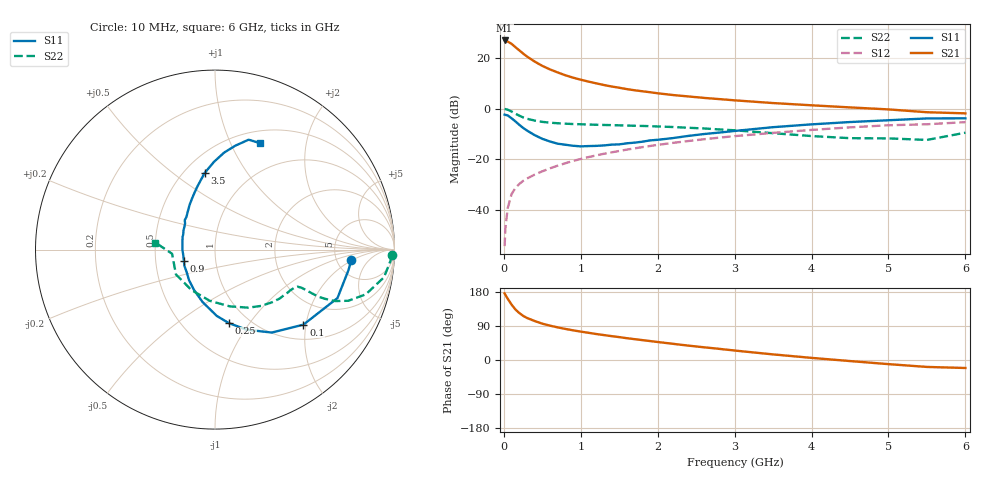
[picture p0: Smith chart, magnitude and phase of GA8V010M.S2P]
! Infineon Technologies  Discrete & RF Semiconductors
! BF775
! Si NPN RF Bipolar Junction Transistor in SOT23
! VCE = 8 V  IC = 10 mA
! Common Emitter S-Parameters:  May  1996
# GHz  S  MA  R  50
!  f  S11  S21  S12  S22
! GHz  MAG  ANG  MAG  ANG  MAG  ANG  MAG  ANG
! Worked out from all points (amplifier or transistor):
!   36 points, 10 MHz to 6 GHz, reference 50 ohm
!   highest |S21| = 27.0 dB at 10 MHz (marker M1)
!   |S21| within 3 dB of that: start of sweep to 164.1 MHz
!   unconditionally stable (mu >= 1): 623.1 MHz to 2.845 GHz
!   at 250 MHz: K = 0.66, MSG = 25.2 dB, |S12| = -28.6 dB
!   at 1.4 GHz: K = 1.09, MAG = 11.2 dB, |S12| = -17.3 dB
!   at 6 GHz: K = 0.89, MSG = 1.7 dB, |S12| = -5.3 dB
!   S11 on the Smith chart (normalised r, x): 10 MHz: 6.85, -1.86; 100 MHz: 1.35, -1.94; 250 MHz: 0.81, -0.80; 900 MHz: 0.70, -0.09; 3.5 GHz: 0.63, +0.65; 6 GHz: 0.64, +1.29
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0.01  0.7608 -4.3  22.35 175.8  0.0019 88.3  0.9876 -1.8
0.02  0.7528 -8.6  21.92 171.9  0.0042 84.3  0.9791 -3.8
0.05  0.7338 -21.6  21.27 161.8  0.0107 80.4  0.9541 -9.3
0.1  0.6462 -40.3  19.17 146.3  0.0203 71.3  0.8768 -16.5
0.15  0.5602 -55.6  16.48 133.4  0.0269 66.9  0.7955 -21.0
0.2  0.48 -68.4  14.26 124.1  0.0322 64.5  0.728 -23.2
0.25  0.4168 -79.3  12.34 116.6  0.0371 63.0  0.6717 -24.1
0.3  0.3695 -88.5  10.78 111.0  0.0414 63.1  0.6318 -24.5
0.4  0.2996 -103.5  8.558 102.9  0.0494 63.0  0.5808 -24.2
0.5  0.253 -117.7  7.018 95.9  0.0575 64.2  0.5474 -23.9
0.6  0.2236 -130.3  5.977 90.6  0.0659 65.1  0.5278 -23.8
0.7  0.2026 -140.8  5.201 86.1  0.0745 65.7  0.514 -24.0
0.8  0.1931 -151.9  4.573 82.0  0.0831 65.5  0.5037 -24.2
0.9  0.1844 -160.1  4.102 78.3  0.0922 65.7  0.4963 -24.9
1.1  0.1817 -179.9  3.432 71.8  0.11 65.7  0.4849 -26.8
1.3  0.1871 165.8  2.938 65.8  0.1279 64.9  0.4754 -28.8
1.6  0.2062 148.2  2.434 57.5  0.1548 63.1  0.4624 -32.8
2.2  0.2617 125.3  1.858 42.7  0.2103 58.3  0.4328 -42.7
3.5  0.43 97.8  1.29 14.8  0.3319 44.7  0.3268 -75.4
4.5  0.5431 84.6  1.058 -2.8  0.4264 32.4  0.2604 -120.7
5.5  0.6403 73.0  0.849 -18.3  0.4911 17.3  0.2403 -174.5
6  0.644 67.3  0.807 -21.1  0.5403 13.3  0.3344 173.3
